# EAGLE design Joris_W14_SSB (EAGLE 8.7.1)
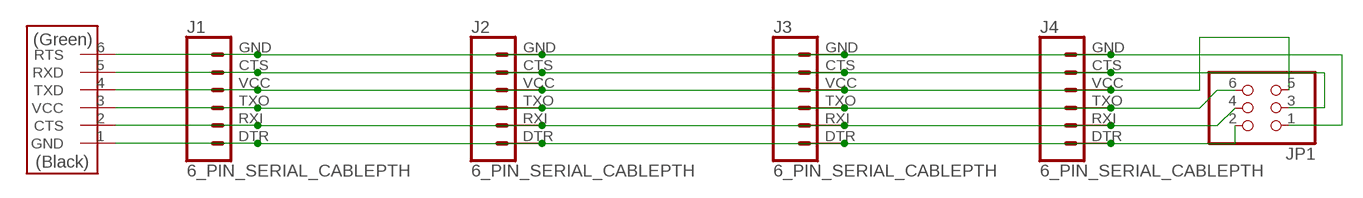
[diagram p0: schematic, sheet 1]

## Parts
J1  6_PIN_SERIAL_CABLEPTH  [FTDI_BASIC]
J2  6_PIN_SERIAL_CABLEPTH  [FTDI_BASIC]
J3  6_PIN_SERIAL_CABLEPTH  [FTDI_BASIC]
J4  6_PIN_SERIAL_CABLEPTH  [FTDI_BASIC]
JP1  PINHD-2X3-SMD  [2X03SMD]
U$1  FTDI-SMD-HEADER  [1X06SMD]

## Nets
N$1: J1.GND J2.GND J3.GND J4.GND JP1.1 U$1.6(RTS)
N$2: J1.CTS J2.CTS J3.CTS J4.CTS JP1.3 U$1.5(RXD)
N$3: J1.VCC J2.VCC J3.VCC J4.VCC JP1.5 U$1.4(TXD)
N$4: J1.TXO J2.TXO J3.TXO J4.TXO JP1.6 U$1.3(VCC)
N$5: J1.RXI J2.RXI J3.RXI J4.RXI JP1.4 U$1.2(CTS)
N$6: J1.DTR J2.DTR J3.DTR J4.DTR JP1.2 U$1.1(GND)

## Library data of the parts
J1-J4 = SparkFun-Connectors:6_PIN_SERIAL_CABLE: 6-pin header connection for use with the "FTDI BASIC" pinout - CABLE SIDE. Also known as "Arduino Serial Program Header". This is used on a design to provide a 6-pin connection point for serial communication usually from a USB cable (D+/D-) to these headers (RX/TX). It also has the remaining pins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
JP1 = fab:PINHD-2X3-SMD: PIN HEADER
U$1 = fab:FTDI-SMD-HEADER

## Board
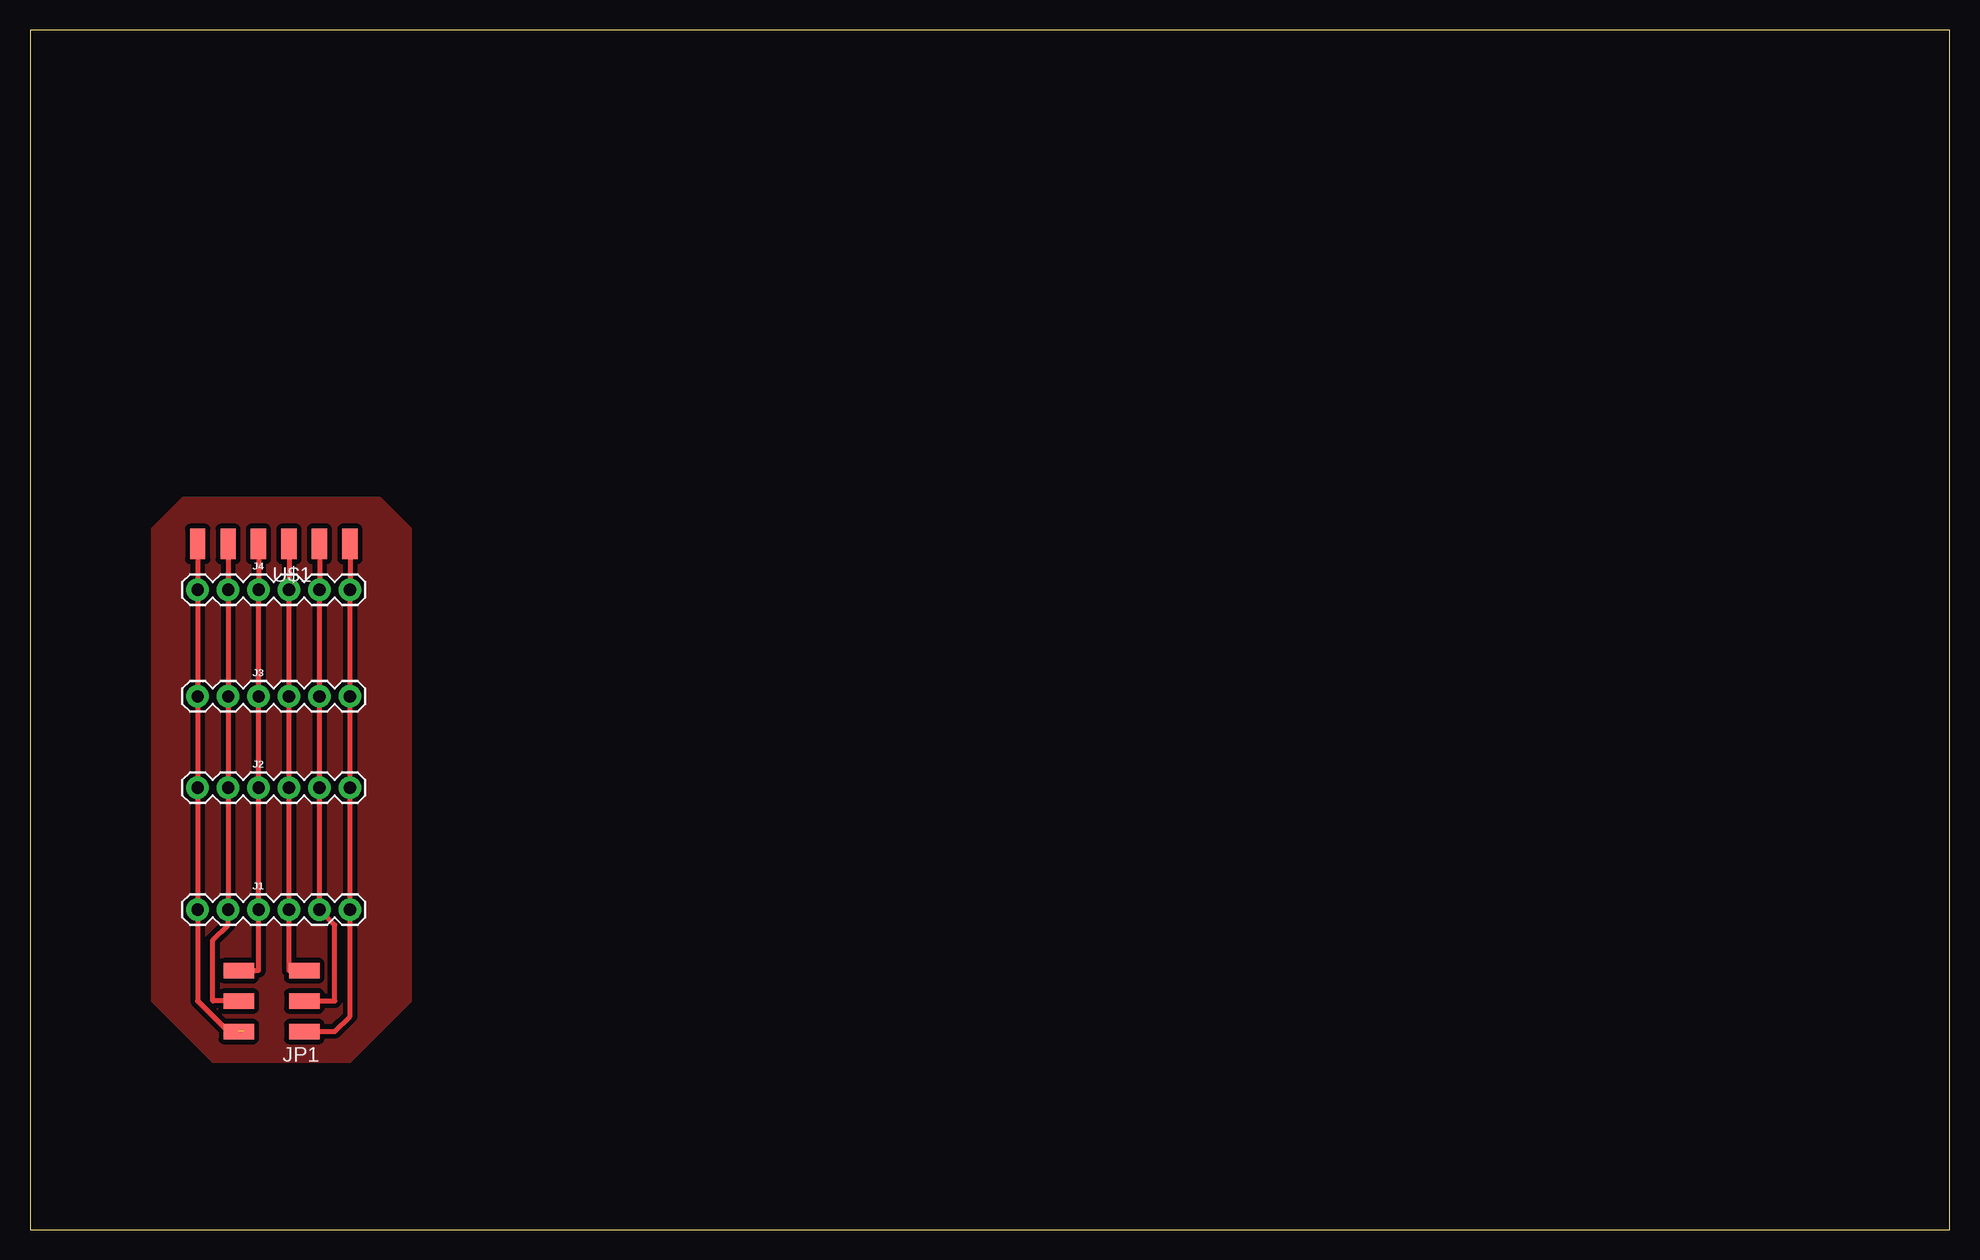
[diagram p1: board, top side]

Size 160 x 100 mm. Coordinates in mm from the lower left corner, seen from the top.
Outline: 0,0 160,0 160,100 0,100 0,0
Copper layers (1*16): Top 0.035mm / dielectric 1.5mm / Bottom 0.035mm
Design rules "default *": minimum track width 6mil, minimum drill 0.35mm, track to track 16mil, track to pad 16mil, pad to pad 16mil, via to via 16mil, smd to smd 16mil, copper to edge 40mil, drill to drill 6mil, minimum pad ring 10mil, minimum via ring 8mil, stop-mask expansion 4mil, vias tented up to drill 0mil, thermal gap 10mil

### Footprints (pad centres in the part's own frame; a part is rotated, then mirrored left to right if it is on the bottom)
FTDI_BASIC = drill 1.016 pad 1.88: CTS 10.16,0; DTR 0,0; GND 12.7,0; RXI 2.54,0; TXO 5.08,0; VCC 7.62,0
2X03SMD = smd 2.54 x 1.27: 1 -2.54,2.54; 2 2.92,2.54; 3 -2.54,0; 4 2.92,0; 5 -2.54,-2.54; 6 2.92,-2.54
1X06SMD = smd 2.54 x 1.27: 1 0,6.35; 2 0,3.81; 3 0,1.27; 4 0,-1.27; 5 0,-3.81; 6 0,-6.35

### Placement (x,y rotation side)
J1  13.97,26.67 0 top
J2  13.97,36.83 0 top
J3  13.97,44.45 0 top
J4  13.97,53.34 0 top
JP1  20.32,19.05 180 top
U$1  20.32,57.15 90 top

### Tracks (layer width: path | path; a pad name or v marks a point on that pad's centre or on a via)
N$1
  Top 0.406: JP1.1 25.4,16.51 26.67,17.78 J1.GND J2.GND J3.GND J4.GND U$1.6
N$2
  Top 0.406: JP1.3 25.4,19.05 25.4,25.4 J1.CTS J2.CTS J3.CTS J4.CTS U$1.5
N$3
  Top 0.406: JP1.5 21.59,21.59 J1.VCC J2.VCC J3.VCC J4.VCC U$1.4
N$4
  Top 0.406: JP1.6 19.05,21.59 J1.TXO J2.TXO J3.TXO J4.TXO U$1.3
N$5
  Top 0.406: JP1.4 15.24,19.05 15.24,24.13 16.51,25.4 J1.RXI J2.RXI J3.RXI J4.RXI U$1.2
N$6  (1 unrouted)
  Top 0.406: 17.78,16.51 16.51,16.51 13.97,19.05 J1.DTR J2.DTR J3.DTR J4.DTR U$1.1
N$7
  pour Top: 12.7,60.96 10.16,58.42 10.16,22.86 10.16,19.05 15.24,13.97 26.67,13.97 31.75,19.05 31.75,58.42 29.21,60.96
